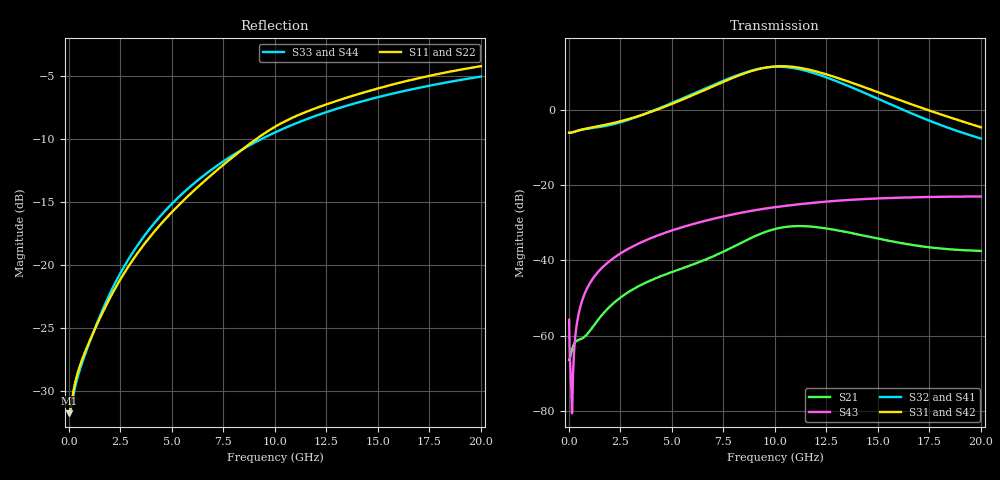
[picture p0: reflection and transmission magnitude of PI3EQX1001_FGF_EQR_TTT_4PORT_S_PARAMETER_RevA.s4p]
! NPort=4 DATA=2000 NOISE=0 GROUPDELAY=0 COMPLEX_DATAFORMAT=POLAR
! NumOfBlock=1 NumOfParam=0
! .MODEL Smodel S TSTONEFILE=PI3EQX1001_FGF_EQR_TTT_4PORT_S_PARAMETER_RevA.s4p TYPE=S
!  -- The above .MODEL line can be used for the S element in the netlist.
! The s parameter is extracted from the linear redriver, it is not bi-directional; only s(4,1)s(4,2) and s(3,1)s(3,2)
! should be the insertion loss
!Port definition:
!Port1 = input+
!Port2 = input¨C
!Port3 = output+
!Port4 = output-
# Hz S MA R  50
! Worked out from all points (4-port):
!   2000 points, 10 MHz to 20 GHz, reference 50 ohm
!   strongest paths, dB at 10 MHz, 5.01 GHz, 10.01 GHz, 15.01 GHz, 20 GHz:
!     S31: -6.1, 1.6, 11.5, 4.7, -4.6
!     S42: -6.1, 1.6, 11.5, 4.7, -4.6
!     S32: -6.1, 1.9, 11.4, 2.9, -7.6
!     S41: -6.1, 1.8, 11.4, 2.9, -7.6
!     S43: -55.8, -32.0, -25.9, -23.5, -23.0
!     S21: -66.4, -43.1, -31.6, -34.2, -37.5
!   lowest |S11| = -31.7 dB at 10 MHz (marker M1), VSWR 1.05, Z = 47.5 - j0.063 ohm
!   |S11| at or under -10 dB: start of sweep to 9.11 GHz
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1e7  0.02591 -178.5  0.0004922 2.7  3.669e-05 -0.2  4.787e-05 -0.1
     0.0004763 2.9  0.02597 -178.7  4.577e-05 -0.2  5.994e-05 -0.1
     0.496 -0.4  0.4959 179.7  0.02616 178.4  0.001615 -59.2
     0.4957 179.7  0.4957 -0.3  0.001626 -58.9  0.02612 178.4
7.29e9  0.2414 -106.1  0.01159 77.9  2.163e-05 -30.9  3.209e-05 -29.7
        0.01229 76.2  0.2395 -106.0  2.884e-05 -25.4  3.968e-05 -25.1
        2.225 -58.9  2.306 126.6  0.2508 -112.2  0.03726 54.6
        2.298 126.7  2.223 -58.8  0.03722 54.7  0.2506 -112.2
9.28e9  0.3234 -108.2  0.02148 61.1  1.96e-05 -27.4  3.352e-05 -33.8
        0.02245 59.4  0.3212 -108.2  3.089e-05 -26.4  3.751e-05 -23.7
        3.512 -114.5  3.533 70.7  0.3136 -115.0  0.04762 41.9
        3.518 70.9  3.51 -114.5  0.04762 41.9  0.3134 -115.0
1.094e10  0.3862 -112.7  0.02737 30.4  2.217e-05 -20.7  3.458e-05 -46.3
          0.0285 29.1  0.3833 -112.7  3.246e-05 -37.8  4.037e-05 -21.4
          3.705 -172.5  3.568 13.1  0.3617 -117.7  0.05479 31.0
          3.553 13.3  3.702 -172.5  0.05476 30.9  0.3614 -117.7
1.328e10  0.4545 -118.0  0.02335 -3.4  2.99e-05 -37.4  2.956e-05 -68.6
          0.02438 -4.6  0.4507 -118.1  2.759e-05 -57.9  4.762e-05 -33.8
          2.524 117.7  2.232 -54.6  0.4226 -121.6  0.06287 15.9
          2.221 -54.2  2.521 117.7  0.06276 15.9  0.4226 -121.6
1.582e10  0.5213 -122.8  0.01672 -17.8  2.939e-05 -71.0  2.098e-05 -98.3
          0.01761 -19.2  0.517 -122.8  1.849e-05 -82.8  4.419e-05 -57.2
          1.422 62.1  1.117 -104.4  0.4796 -125.5  0.06786 0.1
          1.112 -103.8  1.42 62.1  0.06778 0.1  0.4792 -125.5
2e10  0.6131 -130.1  0.01281 -15.6  1.625e-05 -146.7  1.357e-05 145.3
      0.01338 -18.5  0.6077 -130.2  8.775e-06 127.9  1.932e-05 -95.8
      0.5867 -4.5  0.4155 -150.7  0.5577 -131.1  0.07058 -23.4
      0.4157 -149.8  0.5856 -4.5  0.07054 -23.4  0.5576 -131.1
